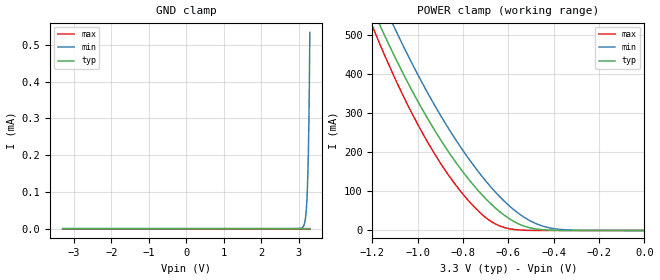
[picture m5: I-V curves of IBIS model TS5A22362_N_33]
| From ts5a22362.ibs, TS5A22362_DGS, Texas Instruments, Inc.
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[Model]   TS5A22362_N_33
Model_type  Terminator
| variable   typ   min   max
C_comp   70.34pF   65.13pF   77.36pF
| C_tri-state   70.34pF   65.13pF   77.36pF
[Temperature Range]   40   100   -40
| Ambient temperature   25   85   -40
[Voltage range]   3.3   3   3.6
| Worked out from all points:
|   POWER clamp passes 1 mA (typ) near -0.42 V on its own axis
[GND Clamp]
| TS5A22362_N_33
|   Voltage   I(typ)   I(min)   I(max)
-3.3V     -1.239nA   -130.3nA   -201pA
3.1V      768.9pA    2.768uA    30.84pA
3.15V     782.2pA    11.33uA    32.32pA
3.185V    797.5pA    29.57uA    33.34pA
3.21V     819.8pA    57.46uA    34.07pA
3.235V    869.8pA    109.6uA    34.8pA
3.255V    959pA      180.9uA    35.38pA
3.27V     1.087nA    261.4uA    35.81pA
3.28V     1.224nA    332.7uA    36.1pA
3.285V    1.314nA    374.9uA    36.24pA
3.295V    1.558nA    475uA      36.53pA
3.3V      1.721nA    534uA      36.67pA
[POWER Clamp]
| TS5A22362_N_33
|   Voltage   I(typ)   I(min)   I(max)
-3.3V     5.424A     5.458A     5.997A
-1.21V    581.2mA    657.9mA    537mA
-1.19V    554.9mA    631mA      508.5mA
-1.165V   522.7mA    597.9mA    473.8mA
-1.105V   448.7mA    521.8mA    394.8mA
-995mV    325.6mA    393.6mA    266.1mA
-890mV    223.8mA    285.5mA    163.6mA
-770mV    127.1mA    179.4mA    72.12mA
-670mV    64.15mA    106.4mA    20.83mA
-555mV    16.83mA    43.51mA    1.406mA
-445mV    1.756mA    10.5mA     34.82uA
0V        0A         0A         0A
